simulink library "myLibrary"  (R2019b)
settings: Solver=VariableStepAuto  StartTime=0.0  StopTime=10.0  RelTol=1e-3
undefined symbols (not defined in the file or in its folder): batt_delay, Calculation, cap_1ph, cap_3ph, Complex, Current, Dynamic, EV, ev_charger, EV_ID, ev_num, gcbh, Iabc, Load, max_charge_1ph, max_charge_3ph, max_disch_1ph, max_disch_3ph, MV_LV_transf, myLibrary, phase, Phase, Phasor, rated_1ph, rated_3ph, Single, SoC_init, SPDL, sps_rtmsupport, Tr_capacity, Tstep, Vabc, Vnom, yes
libraries: powerlib x163, $bdroot x13, spsVIMeasurementModel x3, simulink x2, powerlib_meascontrol x1
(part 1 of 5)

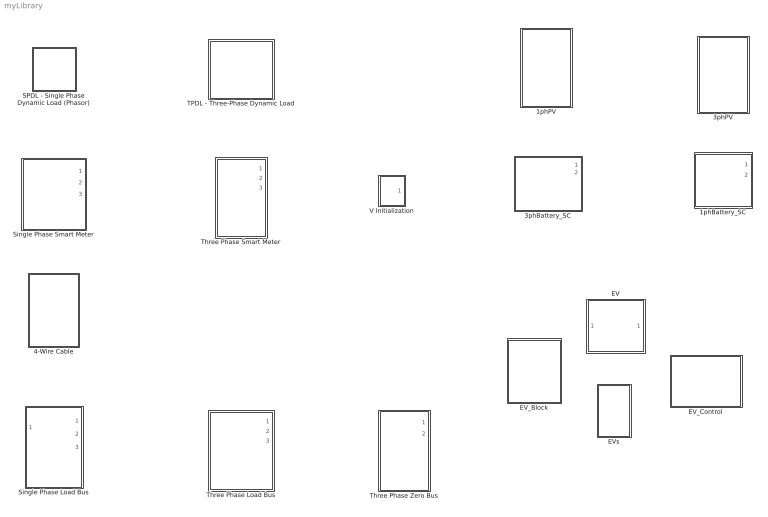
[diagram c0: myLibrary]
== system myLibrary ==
  1phBattery_SC : Subsystem  mask{Ecap=cap_1ph, Sn=rated_1ph, SoC=SoC_init, Pch_max=max_charge_1ph, Pdisc_max=max_disch_1ph, ch_delay=batt_delay, Phase=phase}
      mask prompts: Ecap "Capacity [kWh]"; Sn "Rated power [kVA]"; SoC "Initial SoC [%]"; Pch_max "Max charging rate [kW]"; Pdisc_max "Max discharge rate [kW]"; ch_delay "Charging delay [give integer multiple of time step]"; Phase "Connected Phase [1,2,3]"
      mask help: A 3phase battery system operating at 'self-consumption' mode
  1phPV : Subsystem  mask{Load_Profile=0, Phase=0, Capacity=0}
      mask prompts: Load_Profile "PV Profile"; Phase "Phase (A=1, B=2, C=3)"; Capacity "Capacity [kWp]"
  3phBattery_SC : Subsystem  mask{Ecap=cap_3ph, Sn=rated_3ph, SoC=SoC_init, Pch_max=max_charge_3ph, Pdisc_max=max_disch_3ph, ch_delay=batt_delay}
      mask prompts: Ecap "Capacity [kWh]"; Sn "Rated power [kVA]"; SoC "Initial SoC [%]"; Pch_max "Max charging rate [kW]"; Pdisc_max "Max discharge rate [kW]"; ch_delay "Charging delay [give integer multiple of time step]"
      mask help: A 3phase battery system operating at 'self-consumption' mode
  3phPV : Subsystem  mask{Load_Profile=0, Capacity=0}
      mask prompts: Load_Profile "PV Profile"; Capacity "Capacity [kWp]"
  4-Wire Cable : Subsystem  AncestorBlock=myLibrary/Three Phase Smart Meter  mask{R=0, L=0, C=0, Length=0}
      mask prompts: Length "Length (km)"
  EV : Subsystem  AncestorBlock=myLibrarya/EV  mask{Phase=1, EV_id=EV_ID}
      mask prompts: Phase "Connected Phase [1,2,3]"; EV_id "EV ID"
      mask help: Single Phase EV
  EV_Block : Subsystem  AncestorBlock=myLibrary/EV_Block  InitFcn=|
      | EV_num=20
      | Phase=[5,5,10];
      | ID_first_EV=1;
  EV_Control : Subsystem  AncestorBlock=myLibrary/EV_Control  InitFcn=ev_control_init
  EVs : Subsystem  mask{EV_ID=18, Phase=1}
      mask prompts: EV_ID "EV ID"
      mask init:
      | data_EV=sprintf('EV_num_%d',EV_ID);
      | set_param([gcb '/EVinfo'],'GotoTag',data_EV);
      | 
      | data_EV=sprintf('EV_cont_%d',EV_ID);
      | set_param([gcb '/EVcont'],'GotoTag',data_EV);
  SPDL - Single Phase Dynamic Load (Phasor) : Subsystem  mask(Single-Phase Dynamic Load){Load_Profile=0, Phase=0}
      mask prompts: Phase "Phase [A=1, B=2, C=3]"
      mask help: Single Phase Dynamic Load. The Load Profile is given by an external file.
  Single Phase Load Bus : Subsystem
  Single Phase Smart Meter : Subsystem
  TPDL - Three-Phase Dynamic Load : Subsystem  mask{Load_Profile=0}
  Three Phase Load Bus : Subsystem
  Three Phase Smart Meter : Subsystem
  Three Phase Zero Bus : Subsystem
  V Initialization : Subsystem

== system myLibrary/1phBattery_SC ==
  Constant7 : Constant  Value=0
  Pbatt_SoC : Subsystem
  SPDL2 : Subsystem  mask(Single-Phase Dynamic Load){Phase=Phase}
      mask prompts: Phase "Phase [A=1, B=2, C=3]"
      mask help: Single Phase Dynamic Load. The Load Profile is given by an external file.
  Single Phase Smart Meter : Subsystem
  P : PMIOPort  Tag=PMCPort  Side=Left
  N : PMIOPort  Tag=PMCPort  Port=2  Side=Left
  p : PMIOPort  Port=3  Side=Right
  n : PMIOPort  Port=4  Side=Right
  Pbatt : Outport
  SoC : Outport  Port=2
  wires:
  Constant7/1 -> [Q]
  [Q] -> SPDL2/2(Q)
  [P] -> SPDL2/1(P)
  Single Phase Smart Meter/1(Pout) -> [Pnet]
  [Pnet] -> Pbatt_SoC/1(Pn)
  Pbatt_SoC/1(SoC) -> SoC/1
  Pbatt_SoC/2(Pbatt) -> [P], Pbatt/1
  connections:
  p/RConn1 -- Single Phase Smart Meter/RConn1
  n/RConn1 -- Single Phase Smart Meter/RConn2
  P/RConn1 -- SPDL2/LConn1 -- Single Phase Smart Meter/LConn1
  N/RConn1 -- Single Phase Smart Meter/LConn2 -- SPDL2/LConn2

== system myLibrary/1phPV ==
  1Ph PV : $bdroot/3phPV/1Ph PV  Load_Profile=Load_Profile  Phase=Phase  Capacity=Capacity
  Voltage Measurement1 : powerlib/Measurements/Voltage Measurement  PhasorSimulation=off  OutputType=Complex  PSBequivalent=0
  Phase : PMIOPort  Tag=PMCPort  Side=Left
  N : PMIOPort  Tag=PMCPort  Port=2  Side=Left
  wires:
  Voltage Measurement1/1 -> 1Ph PV/1
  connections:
  Phase/RConn1 -- Voltage Measurement1/LConn1 -- 1Ph PV/LConn1
  N/RConn1 -- Voltage Measurement1/LConn2 -- 1Ph PV/LConn2

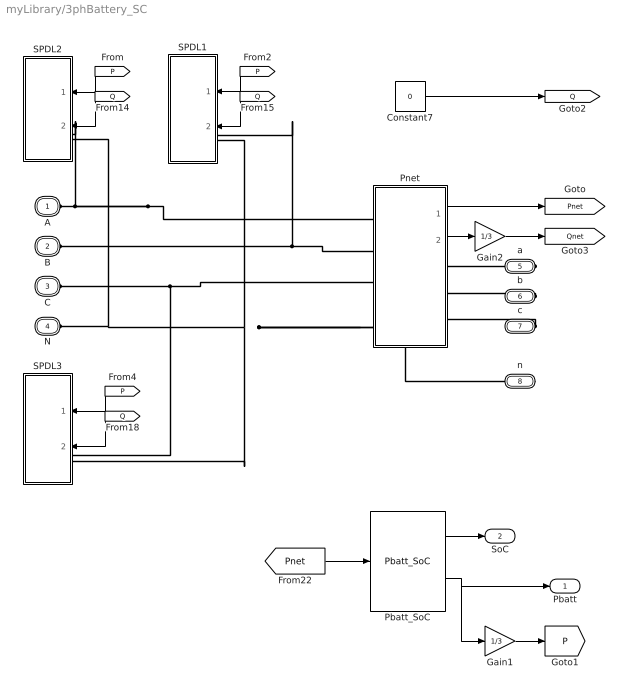
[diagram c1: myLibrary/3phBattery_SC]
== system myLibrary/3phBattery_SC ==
  Constant7 : Constant  Value=0
  Gain1 : Gain  Gain=1/3
  Gain2 : Gain  Gain=1/3
  Pbatt_SoC : $bdroot/1phBattery_SC/Pbatt_SoC  SystemSampleTime=-1  Latency=0  AutoFrameSizeCalculation=off
  Pnet : Subsystem
  SPDL1 : Subsystem  mask(Single-Phase Dynamic Load){Phase=2}
      mask prompts: Phase "Phase [A=1, B=2, C=3]"
      mask help: Single Phase Dynamic Load. The Load Profile is given by an external file.
  SPDL2 : Subsystem  mask(Single-Phase Dynamic Load){Phase=1}
      mask prompts: Phase "Phase [A=1, B=2, C=3]"
      mask help: Single Phase Dynamic Load. The Load Profile is given by an external file.
  SPDL3 : Subsystem  mask(Single-Phase Dynamic Load){Phase=3}
      mask prompts: Phase "Phase [A=1, B=2, C=3]"
      mask help: Single Phase Dynamic Load. The Load Profile is given by an external file.
  A : PMIOPort  Tag=PMCPort  Side=Left
  B : PMIOPort  Tag=PMCPort  Port=2  Side=Left
  C : PMIOPort  Tag=PMCPort  Port=3  Side=Left
  N : PMIOPort  Tag=PMCPort  Port=4  Side=Left
  a : PMIOPort  Port=5  Side=Right
  b : PMIOPort  Port=6  Side=Right
  c : PMIOPort  Port=7  Side=Right
  n : PMIOPort  Port=8  Side=Right
  Pbatt : Outport
  SoC : Outport  Port=2
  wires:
  [P] -> SPDL3/1(P)
  [Q] -> SPDL3/2(Q)
  [Q] -> SPDL2/2(Q)
  Gain2/1 -> [Qnet]
  [P] -> SPDL2/1(P)
  Pnet/1(Pnet) -> [Pnet]
  Constant7/1 -> [Q]
  [Pnet] -> Pbatt_SoC/1
  Gain1/1 -> [P]
  Pbatt_SoC/1 -> SoC/1
  Pbatt_SoC/2 -> Pbatt/1, Gain1/1
  [P] -> SPDL1/1(P)
  [Q] -> SPDL1/2(Q)
  Pnet/2(Qnet) -> Gain2/1
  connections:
  c/RConn1 -- Pnet/RConn3
  b/RConn1 -- Pnet/RConn2
  Pnet/RConn1 -- a/RConn1
  N/RConn1 -- SPDL2/LConn2 -- Pnet/LConn4 -- n/RConn1 -- SPDL3/LConn2 -- SPDL1/LConn2
  B/RConn1 -- SPDL1/LConn1 -- Pnet/LConn2
  C/RConn1 -- Pnet/LConn3 -- SPDL3/LConn1
  A/RConn1 -- SPDL2/LConn1 -- Pnet/LConn1

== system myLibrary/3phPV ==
  1Ph PV : Subsystem  mask{Load_Profile=Load_Profile, Phase=1, Capacity=Capacity/3}
      mask prompts: Load_Profile "PV Profile"; Capacity "Capacity [kWp]"
  1Ph PV1 : $bdroot/3phPV/1Ph PV  Load_Profile=Load_Profile  Phase=2  Capacity=Capacity/3
  1Ph PV2 : $bdroot/3phPV/1Ph PV  Load_Profile=Load_Profile  Phase=3  Capacity=Capacity/3
  Ground2 : powerlib/Elements/Ground  LConnTagsString=a
  Voltage Measurement : powerlib/Measurements/Voltage Measurement  PhasorSimulation=off  OutputType=Complex  PSBequivalent=0
  Voltage Measurement1 : powerlib/Measurements/Voltage Measurement  PhasorSimulation=off  OutputType=Complex  PSBequivalent=0
  Voltage Measurement2 : powerlib/Measurements/Voltage Measurement  PhasorSimulation=off  OutputType=Complex  PSBequivalent=0
  A : PMIOPort  Tag=PMCPort  Side=Left
  B : PMIOPort  Tag=PMCPort  Port=2  Side=Left
  C : PMIOPort  Tag=PMCPort  Port=3  Side=Left
  N : PMIOPort  Tag=PMCPort  Port=4  Side=Left
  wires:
  Voltage Measurement2/1 -> 1Ph PV/1(Vp)
  Voltage Measurement/1 -> 1Ph PV1/1
  Voltage Measurement1/1 -> 1Ph PV2/1
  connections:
  1Ph PV1/LConn2 -- 1Ph PV/LConn2 -- 1Ph PV2/LConn2 -- N/RConn1
  Voltage Measurement1/LConn1 -- 1Ph PV2/LConn1 -- C/RConn1
  Voltage Measurement/LConn1 -- 1Ph PV1/LConn1 -- B/RConn1
  Voltage Measurement2/LConn1 -- 1Ph PV/LConn1 -- A/RConn1
  Ground2/LConn1 -- Voltage Measurement1/LConn2 -- Voltage Measurement/LConn2 -- Voltage Measurement2/LConn2

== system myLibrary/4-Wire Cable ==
  Cag : powerlib/Elements/Series RLC Branch  LConnTagsString=__new0  RConnTagsString=__new0  BranchType=C  Resistance=1  Inductance=1e-3  SetiL0=off  InitialCurrent=0  Capacitance=C(1,1)*Length/2  Setx0=off  InitialVoltage=0  Measurements=None
  Cag1 : powerlib/Elements/Series RLC Branch  LConnTagsString=__new0  RConnTagsString=__new0  BranchType=C  Resistance=1  Inductance=1e-3  SetiL0=off  InitialCurrent=0  Capacitance=C(1,1)*Length/2  Setx0=off  InitialVoltage=0  Measurements=None
  Cbg : powerlib/Elements/Series RLC Branch  LConnTagsString=__new0  RConnTagsString=__new0  BranchType=C  Resistance=1  Inductance=1e-3  SetiL0=off  InitialCurrent=0  Capacitance=C(1,1)*Length/2  Setx0=off  InitialVoltage=0  Measurements=None
  Cbg1 : powerlib/Elements/Series RLC Branch  LConnTagsString=__new0  RConnTagsString=__new0  BranchType=C  Resistance=1  Inductance=1e-3  SetiL0=off  InitialCurrent=0  Capacitance=C(1,1)*Length/2  Setx0=off  InitialVoltage=0  Measurements=None
  Ccg : powerlib/Elements/Series RLC Branch  LConnTagsString=__new0  RConnTagsString=__new0  BranchType=C  Resistance=1  Inductance=1e-3  SetiL0=off  InitialCurrent=0  Capacitance=C(1,1)*Length/2  Setx0=off  InitialVoltage=0  Measurements=None
  Ccg1 : powerlib/Elements/Series RLC Branch  LConnTagsString=__new0  RConnTagsString=__new0  BranchType=C  Resistance=1  Inductance=1e-3  SetiL0=off  InitialCurrent=0  Capacitance=C(1,1)*Length/2  Setx0=off  InitialVoltage=0  Measurements=None
  Cng : powerlib/Elements/Series RLC Branch  LConnTagsString=__new0  RConnTagsString=__new0  BranchType=C  Resistance=1  Inductance=1e-3  SetiL0=off  InitialCurrent=0  Capacitance=C(2,1)*Length/2  Setx0=off  InitialVoltage=0  Measurements=None
  Cng1 : powerlib/Elements/Series RLC Branch  LConnTagsString=__new0  RConnTagsString=__new0  BranchType=C  Resistance=1  Inductance=1e-3  SetiL0=off  InitialCurrent=0  Capacitance=C(2,1)*Length/2  Setx0=off  InitialVoltage=0  Measurements=None
  Ground1 : powerlib/Elements/Ground  LConnTagsString=a
  Ground2 : powerlib/Elements/Ground  LConnTagsString=a
  Mutual Inductance : powerlib/Elements/Mutual Inductance  LConnTagsString=a|b|c|L4  RConnTagsString=A|B|C|R4  TypeOfMutual=Generalized mutual inductance  NumberOfWindings=4  SelfImpedance1=[1.1 1.1e-03]  SelfImpedance2=[ 1.1 1.1e-03]  ThreeWindings=on  SelfImpedance3=[ 1.1 1.1e-03]  MutualImpedance=[1.0 1.0e-03]  InductanceMatrix=L*Length  ResistanceMatrix=R*Length  Measurements=None
  A : PMIOPort  Side=Left
  B : PMIOPort  Port=2  Side=Left
  C : PMIOPort  Port=3  Side=Left
  N : PMIOPort  Port=4  Side=Left
  a : PMIOPort  Port=5  Side=Right
  b : PMIOPort  Port=6  Side=Right
  c : PMIOPort  Port=7  Side=Right
  n : PMIOPort  Port=8  Side=Right
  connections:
  A/RConn1 -- Mutual Inductance/LConn1 -- Cag/LConn1
  Mutual Inductance/RConn1 -- Cag1/LConn1 -- a/RConn1
  B/RConn1 -- Cbg/LConn1 -- Mutual Inductance/LConn2
  Mutual Inductance/RConn2 -- Cbg1/LConn1 -- b/RConn1
  C/RConn1 -- Ccg/LConn1 -- Mutual Inductance/LConn3
  c/RConn1 -- Ccg1/LConn1 -- Mutual Inductance/RConn3
  N/RConn1 -- Cng/LConn1 -- Mutual Inductance/LConn4
  n/RConn1 -- Cng1/LConn1 -- Mutual Inductance/RConn4
  Cag/RConn1 -- Ground2/LConn1 -- Cng/RConn1 -- Ccg/RConn1 -- Cbg/RConn1
  Cag1/RConn1 -- Ground1/LConn1 -- Cng1/RConn1 -- Ccg1/RConn1 -- Cbg1/RConn1

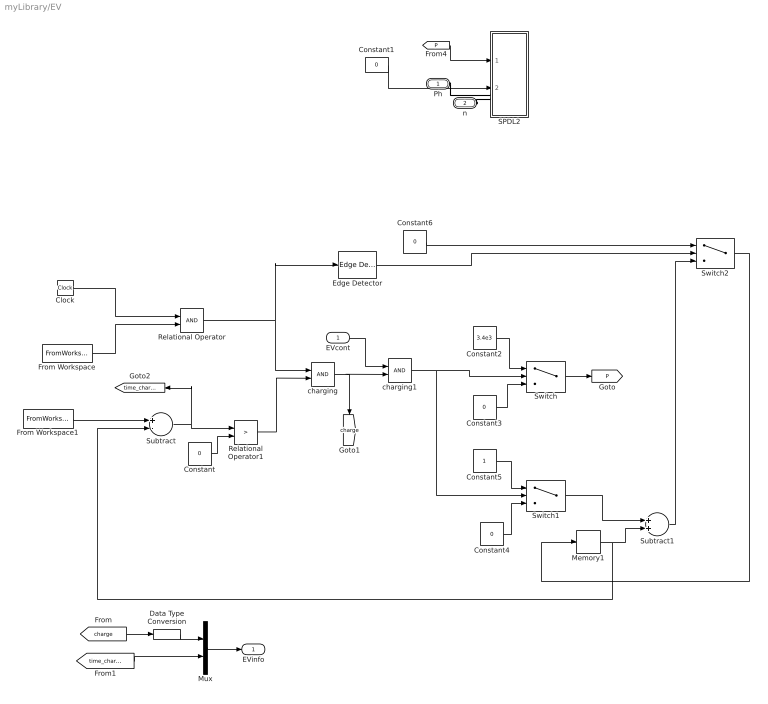
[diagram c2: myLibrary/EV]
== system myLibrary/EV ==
  EVcont : Inport
  Clock : Clock
  Constant{,1,3..4,6} (5 alike) : Constant  Value=0
  Constant2 : Constant  Value=3.4e3
  Constant5 : Constant
  Data Type Conversion : DataTypeConversion  OutDataTypeStr=double
  Edge Detector : powerlib_meascontrol/Logic/Edge Detector  model=Falling  ic=0  Ts=0
  From Workspace : FromWorkspace  VariableName=ch_t(EV_id)  Interpolate=off  OutputAfterFinalValue=Holding final value
  From Workspace1 : FromWorkspace  VariableName=needed_time_ch(EV_id)  Interpolate=off  OutputAfterFinalValue=Holding final value
  Memory1 : Memory
  Mux : Mux  Inputs=2
  Relational Operator : RelationalOperator  OutDataTypeStr=boolean  RndMeth=Simplest
  Relational Operator1 : RelationalOperator  Operator=>  OutDataTypeStr=boolean  RndMeth=Simplest
  SPDL2 : Subsystem  AncestorBlock=myLibrary/SPDL - Single Phase Dynamic Load (Phasor)  mask(Single-Phase Dynamic Load){Phase=Phase}
      mask prompts: Phase "Phase [A=1, B=2, C=3]"
      mask help: Single Phase Dynamic Load. The Load Profile is given by an external file.
  Subtract : Sum  Inputs=+-
  Subtract1 : Sum
  Switch : Switch  Criteria=u2 > Threshold
  Switch1 : Switch  Criteria=u2 > Threshold
  Switch2 : Switch  Criteria=u2 > Threshold
  charging : Logic  AllPortsSameDT=off  OutDataTypeStr=boolean
  charging1 : Logic  AllPortsSameDT=off  OutDataTypeStr=boolean
  Ph : PMIOPort  Side=Left
  n : PMIOPort  Port=2  Side=Left
  EVinfo : Outport
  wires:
  Data Type Conversion/1 -> Mux/1
  EVcont/1 -> charging1/1
  charging1/1 -> Switch/2, Switch1/2
  Mux/1 -> EVinfo/1
  [time_charge] -> Mux/2
  [charge] -> Data Type Conversion/1
  Switch2/1 -> Memory1/1
  Subtract1/1 -> Switch2/3
  Constant6/1 -> Switch2/1
  Edge Detector/1 -> Switch2/2
  Memory1/1 -> Subtract1/2, Subtract/2
  Switch1/1 -> Subtract1/1
  Constant5/1 -> Switch1/1
  Constant4/1 -> Switch1/3
  Switch/1 -> [P]
  Constant1/1 -> SPDL2/2(Q)
  [P] -> SPDL2/1(P)
  Constant3/1 -> Switch/3
  Constant2/1 -> Switch/1
  charging/1 -> [charge], charging1/2
  Relational Operator1/1 -> charging/2
  Relational Operator/1 -> charging/1, Edge Detector/1
  From Workspace1/1 -> Subtract/1
  Constant/1 -> Relational Operator1/2
  Subtract/1 -> Relational Operator1/1, [time_charge]
  From Workspace/1 -> Relational Operator/2
  Clock/1 -> Relational Operator/1
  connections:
  n/RConn1 -- SPDL2/LConn2
  Ph/RConn1 -- SPDL2/LConn1

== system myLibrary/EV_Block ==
  Block_EVs : Subsystem  InitFcn=ev_block_init
  A : PMIOPort  Tag=PMCPort  Side=Left
  B : PMIOPort  Tag=PMCPort  Port=2  Side=Left
  C : PMIOPort  Tag=PMCPort  Port=3  Side=Left
  N : PMIOPort  Tag=PMCPort  Port=4  Side=Left
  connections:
  A/RConn1 -- Block_EVs/LConn1
  B/RConn1 -- Block_EVs/LConn2
  C/RConn1 -- Block_EVs/LConn3
  N/RConn1 -- Block_EVs/LConn4

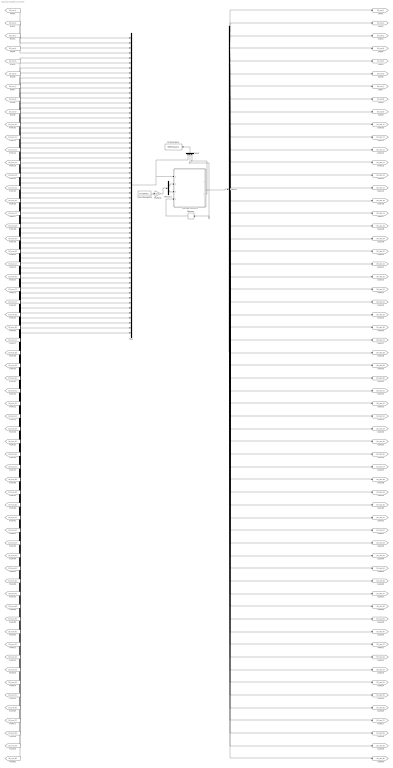
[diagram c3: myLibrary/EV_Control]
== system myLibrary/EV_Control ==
  Demux : Demux  Outputs=ev_num
  Demux1 : Demux  Outputs=2
  From Workspace : FromWorkspace  VariableName=Total_S  SampleTime=0  Interpolate=off  OutputAfterFinalValue=Holding final value
  MATLAB Function : MATLAB Function  TreatAsAtomicUnit=on
  Memory : Memory
  Multiply : Gain  Gain=1/1e3
  Mux : Mux  Inputs=ev_num
  Mux2 : Mux  Inputs=3
  To Workspace : ToWorkspace  VariableName=EVsignals  SaveFormat=Structure With Time  SampleTime=-1
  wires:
  From Workspace/1 -> Multiply/1
  Mux/1 -> MATLAB Function/1(EVsignals), Mux2/1
  MATLAB Function/1(EV_cont_signals) -> Memory/1, Demux/1, Mux2/2
  MATLAB Function/2(k) -> Mux2/3
  Mux2/1 -> To Workspace/1
  Memory/1 -> MATLAB Function/4(were_charging)
  Multiply/1 -> Demux1/1
  Demux1/1 -> MATLAB Function/2(P)
  Demux1/2 -> MATLAB Function/3(Q)
  [EV_num_1] -> Mux/1
  Demux/1 -> [EV_cont_1]
  [EV_num_2] -> Mux/2
  Demux/2 -> [EV_cont_2]
  [EV_num_3] -> Mux/3
  Demux/3 -> [EV_cont_3]
  [EV_num_4] -> Mux/4
  Demux/4 -> [EV_cont_4]
  [EV_num_5] -> Mux/5
  Demux/5 -> [EV_cont_5]
  [EV_num_6] -> Mux/6
  Demux/6 -> [EV_cont_6]
  [EV_num_7] -> Mux/7
  Demux/7 -> [EV_cont_7]
  [EV_num_8] -> Mux/8
  Demux/8 -> [EV_cont_8]
  [EV_num_9] -> Mux/9
  Demux/9 -> [EV_cont_9]
  [EV_num_10] -> Mux/10
  Demux/10 -> [EV_cont_10]
  [EV_num_11] -> Mux/11
  Demux/11 -> [EV_cont_11]
  [EV_num_12] -> Mux/12
  Demux/12 -> [EV_cont_12]
  [EV_num_13] -> Mux/13
  Demux/13 -> [EV_cont_13]
  [EV_num_14] -> Mux/14
  Demux/14 -> [EV_cont_14]
  [EV_num_15] -> Mux/15
  Demux/15 -> [EV_cont_15]
  [EV_num_16] -> Mux/16
  Demux/16 -> [EV_cont_16]
  [EV_num_17] -> Mux/17
  Demux/17 -> [EV_cont_17]
  [EV_num_18] -> Mux/18
  Demux/18 -> [EV_cont_18]
  [EV_num_19] -> Mux/19
  Demux/19 -> [EV_cont_19]
  [EV_num_20] -> Mux/20
  Demux/20 -> [EV_cont_20]
  [EV_num_21] -> Mux/21
  Demux/21 -> [EV_cont_21]
  [EV_num_22] -> Mux/22
  Demux/22 -> [EV_cont_22]
  [EV_num_23] -> Mux/23
  Demux/23 -> [EV_cont_23]
  [EV_num_24] -> Mux/24
  Demux/24 -> [EV_cont_24]
  [EV_num_25] -> Mux/25
  Demux/25 -> [EV_cont_25]
  [EV_num_26] -> Mux/26
  Demux/26 -> [EV_cont_26]
  [EV_num_27] -> Mux/27
  Demux/27 -> [EV_cont_27]
  [EV_num_28] -> Mux/28
  Demux/28 -> [EV_cont_28]
  [EV_num_29] -> Mux/29
  Demux/29 -> [EV_cont_29]
  [EV_num_30] -> Mux/30
  Demux/30 -> [EV_cont_30]
  [EV_num_31] -> Mux/31
  Demux/31 -> [EV_cont_31]
  [EV_num_32] -> Mux/32
  Demux/32 -> [EV_cont_32]
  [EV_num_33] -> Mux/33
  Demux/33 -> [EV_cont_33]
  [EV_num_34] -> Mux/34
  Demux/34 -> [EV_cont_34]
  [EV_num_35] -> Mux/35
  Demux/35 -> [EV_cont_35]
  [EV_num_36] -> Mux/36
  Demux/36 -> [EV_cont_36]
  [EV_num_37] -> Mux/37
  Demux/37 -> [EV_cont_37]
  [EV_num_38] -> Mux/38
  Demux/38 -> [EV_cont_38]
  [EV_num_39] -> Mux/39
  Demux/39 -> [EV_cont_39]
  [EV_num_40] -> Mux/40
  Demux/40 -> [EV_cont_40]
  [EV_num_41] -> Mux/41
  Demux/41 -> [EV_cont_41]
  [EV_num_42] -> Mux/42
  Demux/42 -> [EV_cont_42]
  [EV_num_43] -> Mux/43
  Demux/43 -> [EV_cont_43]
  [EV_num_44] -> Mux/44
  Demux/44 -> [EV_cont_44]
  [EV_num_45] -> Mux/45
  Demux/45 -> [EV_cont_45]
  [EV_num_46] -> Mux/46
  Demux/46 -> [EV_cont_46]
  [EV_num_47] -> Mux/47
  Demux/47 -> [EV_cont_47]
  [EV_num_48] -> Mux/48
  Demux/48 -> [EV_cont_48]
  [EV_num_49] -> Mux/49
  Demux/49 -> [EV_cont_49]
  [EV_num_50] -> Mux/50
  Demux/50 -> [EV_cont_50]
  [EV_num_51] -> Mux/51
  Demux/51 -> [EV_cont_51]
  [EV_num_52] -> Mux/52
  Demux/52 -> [EV_cont_52]
  [EV_num_53] -> Mux/53
  Demux/53 -> [EV_cont_53]
  [EV_num_54] -> Mux/54
  Demux/54 -> [EV_cont_54]
  [EV_num_55] -> Mux/55
  Demux/55 -> [EV_cont_55]
  [EV_num_56] -> Mux/56
  Demux/56 -> [EV_cont_56]
  [EV_num_57] -> Mux/57
  Demux/57 -> [EV_cont_57]
  [EV_num_58] -> Mux/58
  Demux/58 -> [EV_cont_58]
  [EV_num_59] -> Mux/59
  Demux/59 -> [EV_cont_59]
  [EV_num_60] -> Mux/60
  Demux/60 -> [EV_cont_60]

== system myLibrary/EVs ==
  EV2 : $bdroot/EV  Phase=Phase  EV_id=EV_ID
  Ph : PMIOPort  Side=Left
  n : PMIOPort  Port=2  Side=Left
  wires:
  [EV_cont_18] -> EV2/1
  EV2/1 -> [EV_num_18]
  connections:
  EV2/LConn1 -- Ph/RConn1
  EV2/LConn2 -- n/RConn1

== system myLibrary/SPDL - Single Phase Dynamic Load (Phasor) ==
  Breaker : powerlib/Elements/Breaker  InitialState=1  SwitchingTimes=0  External=off  BreakerResistance=0.01  SnubberResistance=1e3  SnubberCapacitance=inf  Measurements=None  MoreParameters=on  NoBreakLoop=off
  Controlled Current Source : powerlib/Electrical Sources/Controlled Current Source  Initialize=on  Source_Type=AC  Amplitude=0  Phase=0  Frequency=50  Measurements=None
  Current Calculation : Subsystem
  Gain : Gain  Gain=sqrt(2)
  Snubber4 : powerlib/Elements/Series RLC Branch  LConnTagsString=__new0  RConnTagsString=__new0  BranchType=R  Resistance=1e6  Inductance=1e-3  SetiL0=off  InitialCurrent=0  Capacitance=1e-6  Setx0=off  InitialVoltage=0  Measurements=None
  Step : Step  Time=0.001  Before=-1  SampleTime=0
  Switch : Switch  Criteria=u2 > Threshold
  V Initialization : $bdroot/V Initialization  SystemSampleTime=-1  Latency=0  AutoFrameSizeCalculation=off
  Voltage Measurement : powerlib/Measurements/Voltage Measurement  PhasorSimulation=off  OutputType=Complex  PSBequivalent=0
  Phase : PMIOPort  Side=Left
  Neutral : PMIOPort  Port=2  Side=Left
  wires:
  Voltage Measurement/1 -> [Vm_c]
  Switch/1 -> Current Calculation/1(Vp)
  Current Calculation/1(Isignal) -> [Icontrol]
  [Icontrol] -> Controlled Current Source/1
  [Vm_c] -> Switch/1
  V Initialization/1 -> Gain/1
  Step/1 -> Switch/2
  Gain/1 -> Switch/3
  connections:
  Voltage Measurement/LConn2 -- Snubber4/RConn1 -- Controlled Current Source/RConn1 -- Neutral/RConn1
  Controlled Current Source/LConn1 -- Breaker/RConn1 -- Voltage Measurement/LConn1 -- Phase/RConn1
  Snubber4/LConn1 -- Breaker/LConn1

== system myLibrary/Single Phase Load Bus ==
  Ph : Inport
  Complex to Magnitude-Angle : ComplexToMagnitudeAngle
  Complex to Magnitude-Angle1 : ComplexToMagnitudeAngle
  Mux3 : Mux  Inputs=2
  Mux4 : Mux  Inputs=2
  Rad->Deg. : Gain  Gain=1/sqrt(2)
  Rad->Deg.1 : Gain  Gain=1/sqrt(2)
  Rad->Deg.2 : Gain  Gain=180/pi
  Rad->Deg.3 : Gain  Gain=180/pi
  Single Phase Smart Meter : $bdroot/Single Phase Smart Meter  SystemSampleTime=-1  Latency=0  AutoFrameSizeCalculation=off
  Subsystem : Subsystem
  Phase : PMIOPort  Tag=PMCPort  Side=Left
  N : PMIOPort  Tag=PMCPort  Port=2  Side=Left
  phase : PMIOPort  Tag=PMCPort  Port=3  Side=Right
  n : PMIOPort  Tag=PMCPort  Port=4  Side=Right
  Vnode : Outport  VectorParamsAs1DForOutWhenUnconnected=off
  Inode : Outport  Port=2  VectorParamsAs1DForOutWhenUnconnected=off
  Lmeas : Outport  Port=3  VectorParamsAs1DForOutWhenUnconnected=off
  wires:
  Single Phase Smart Meter/1 -> Subsystem/1(Vpn)
  Complex to Magnitude-Angle/1 -> Rad->Deg./1
  Rad->Deg.2/1 -> Mux4/2
  Rad->Deg.3/1 -> Mux3/2
  Rad->Deg.1/1 -> Mux3/1
  Complex to Magnitude-Angle1/1 -> Rad->Deg.1/1
  Rad->Deg./1 -> Mux4/1
  Mux4/1 -> Vnode/1
  Subsystem/2("I_pn ") -> Complex to Magnitude-Angle1/1
  Complex to Magnitude-Angle1/2 -> Rad->Deg.3/1
  Complex to Magnitude-Angle/2 -> Rad->Deg.2/1
  Mux3/1 -> Inode/1
  Subsystem/1(V_pn) -> Complex to Magnitude-Angle/1
  Single Phase Smart Meter/2 -> Subsystem/2(Ipn)
  Single Phase Smart Meter/3 -> Lmeas/1
  Ph/1 -> Subsystem/3(Ph)
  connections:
  Phase/RConn1 -- Single Phase Smart Meter/LConn1
  N/RConn1 -- Single Phase Smart Meter/LConn2
  phase/RConn1 -- Single Phase Smart Meter/RConn1
  Single Phase Smart Meter/RConn2 -- n/RConn1

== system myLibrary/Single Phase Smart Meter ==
  Meas : Subsystem
  Phase-Ground Measurements : Subsystem
  Phase-Neutral Measurements : Subsystem
  Phase : PMIOPort  Side=Left
  Neutral : PMIOPort  Port=2  Side=Left
  phase : PMIOPort  Port=3  Side=Right
  neutral : PMIOPort  Port=4  Side=Right
  Vp_Vn : Outport  VectorParamsAs1DForOutWhenUnconnected=off
  Ip_In : Outport  Port=2  VectorParamsAs1DForOutWhenUnconnected=off
  Measurements : Outport  Port=3  VectorParamsAs1DForOutWhenUnconnected=off
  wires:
  Phase-Ground Measurements/2(Ip_In) -> Ip_In/1, Meas/2(Ipn)
  Meas/1(Measurements) -> Measurements/1
  Phase-Ground Measurements/1(Vp_Vn) -> Vp_Vn/1
  Phase-Neutral Measurements/1(Vpn) -> Meas/1(Vpn)
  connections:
  Phase-Ground Measurements/LConn1 -- Phase-Neutral Measurements/LConn1 -- Phase/RConn1
  Neutral/RConn1 -- Phase-Neutral Measurements/LConn2 -- Phase-Ground Measurements/LConn2
  phase/RConn1 -- Phase-Ground Measurements/RConn1
  neutral/RConn1 -- Phase-Ground Measurements/RConn2

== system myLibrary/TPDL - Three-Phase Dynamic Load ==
  SPDL - Single Phase Dynamic Load (Phasor) : Subsystem  mask(Single-Phase Dynamic Load){Load_Profile=Load_Profile, Phase=1}
      mask prompts: Phase "Phase [A=1, B=2, C=3]"
      mask help: Single Phase Dynamic Load. The Load Profile is given by an external file.
  SPDL - Single Phase Dynamic Load (Phasor)1 : Subsystem  mask(Single-Phase Dynamic Load){Load_Profile=Load_Profile, Phase=2}
      mask prompts: Phase "Phase [A=1, B=2, C=3]"
      mask help: Single Phase Dynamic Load. The Load Profile is given by an external file.
  SPDL - Single Phase Dynamic Load (Phasor)2 : Subsystem  mask(Single-Phase Dynamic Load){Load_Profile=Load_Profile, Phase=3}
      mask prompts: Phase "Phase [A=1, B=2, C=3]"
      mask help: Single Phase Dynamic Load. The Load Profile is given by an external file.
  A : PMIOPort  Side=Left
  B : PMIOPort  Port=2  Side=Left
  C : PMIOPort  Port=3  Side=Left
  N : PMIOPort  Port=4  Side=Left
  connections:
  A/RConn1 -- SPDL - Single Phase Dynamic Load (Phasor)/LConn1
  B/RConn1 -- SPDL - Single Phase Dynamic Load (Phasor)1/LConn1
  C/RConn1 -- SPDL - Single Phase Dynamic Load (Phasor)2/LConn1
  N/RConn1 -- SPDL - Single Phase Dynamic Load (Phasor)/LConn2 -- SPDL - Single Phase Dynamic Load (Phasor)1/LConn2 -- SPDL - Single Phase Dynamic Load (Phasor)2/LConn2

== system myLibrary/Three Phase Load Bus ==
  Complex to Magnitude-Angle : ComplexToMagnitudeAngle
  Complex to Magnitude-Angle1 : ComplexToMagnitudeAngle
  Mux3 : Mux  Inputs=2
  Mux4 : Mux  Inputs=2
  Rad->Deg. : Gain  Gain=1/sqrt(2)
  Rad->Deg.1 : Gain  Gain=1/sqrt(2)
  Rad->Deg.2 : Gain  Gain=180/pi
  Rad->Deg.3 : Gain  Gain=180/pi
  Three Phase Smart Meter : $bdroot/Three Phase Smart Meter  SystemSampleTime=-1  Latency=0  AutoFrameSizeCalculation=off
  A : PMIOPort  Tag=PMCPort  Side=Left
  B : PMIOPort  Tag=PMCPort  Port=2  Side=Left
  C : PMIOPort  Tag=PMCPort  Port=3  Side=Left
  N : PMIOPort  Tag=PMCPort  Port=4  Side=Left
  a : PMIOPort  Tag=PMCPort  Port=5  Side=Right
  b : PMIOPort  Tag=PMCPort  Port=6  Side=Right
  c : PMIOPort  Tag=PMCPort  Port=7  Side=Right
  n : PMIOPort  Tag=PMCPort  Port=8  Side=Right
  Vnode : Outport  VectorParamsAs1DForOutWhenUnconnected=off
  Inode : Outport  Port=2  VectorParamsAs1DForOutWhenUnconnected=off
  Lmeas : Outport  Port=3  VectorParamsAs1DForOutWhenUnconnected=off
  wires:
  Three Phase Smart Meter/3 -> Lmeas/1
  Complex to Magnitude-Angle1/1 -> Rad->Deg.1/1
  Complex to Magnitude-Angle1/2 -> Rad->Deg.3/1
  Complex to Magnitude-Angle/2 -> Rad->Deg.2/1
  Mux3/1 -> Inode/1
  Rad->Deg./1 -> Mux4/1
  Mux4/1 -> Vnode/1
  Rad->Deg.3/1 -> Mux3/2
  Rad->Deg.1/1 -> Mux3/1
  Rad->Deg.2/1 -> Mux4/2
  Complex to Magnitude-Angle/1 -> Rad->Deg./1
  Three Phase Smart Meter/1 -> Complex to Magnitude-Angle/1
  Three Phase Smart Meter/2 -> Complex to Magnitude-Angle1/1
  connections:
  A/RConn1 -- Three Phase Smart Meter/LConn1
  B/RConn1 -- Three Phase Smart Meter/LConn2
  C/RConn1 -- Three Phase Smart Meter/LConn3
  N/RConn1 -- Three Phase Smart Meter/LConn4
  a/RConn1 -- Three Phase Smart Meter/RConn1
  Three Phase Smart Meter/RConn2 -- b/RConn1
  Three Phase Smart Meter/RConn3 -- c/RConn1
  Three Phase Smart Meter/RConn4 -- n/RConn1

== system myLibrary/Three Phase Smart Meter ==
  Current Measurement : powerlib/Measurements/Current Measurement  PhasorSimulation=off  OutputType=Complex  PSBequivalent=0
  Ground1 : powerlib/Elements/Ground  LConnTagsString=a
  Mux : Mux  Inputs=2
  Mux1 : Mux  Inputs=2
  Mux2 : Mux  Inputs=3
  Three Phase Smart Meter : Subsystem
  Three-Phase V-I Measurement : Subsystem  AncestorBlock=powerlib/Measurements/Three-Phase V-I Measurement  DialogController=POWERSYS.PowerSysDialog  LoadFcn=|  StartFcn=sps_rtmsupport('StartFcn',gcbh);  StopFcn=sps_rtmsupport('StopFcn',gcbh);  mask(Three-Phase VI Measurement){VoltageMeasurement=phase-to-ground, SetLabelV=off, LabelV=Vabc, Vpu=off, VpuLL=off, CurrentMeasurement=yes, SetLabelI=off, LabelI=Iabc, Ipu=off, Pbase=100e6, Vbase=500e3, OutputType=Complex, PhasorSimulation=off, PSBequivalent=0}
      | if ~strcmp(get_param(bdroot,'BlockDiagramType'),'library')
      |     set_param([gcb,'/Model'],'LinkStatus','restore');
      | end
      | sps_rtmsupport('LoadFcn',gcbh);
      mask prompts: VoltageMeasurement "Voltage measurement"; SetLabelV "Use a label"; LabelV "Signal label  (use a From block to collect this signal)"; Vpu "Voltages in pu,  based on peak value of nominal phase-to-ground voltage"; VpuLL "Voltages in pu,  based on peak value of nominal phase-to-phase  voltage"; CurrentMeasurement "Current measurement"; SetLabelI "Use a label"; LabelI "Signal label  (use a From block to collect this signal)"; Ipu "Currents in pu"; Pbase "Base power ( VA 3 phase)"; Vbase "Nominal voltage used for pu measurement (Vrms phase-phase) :"; OutputType "Output signals in:"; PhasorSimulation "Phasor simulation (internal use)"; PSBequivalent "Equivalent circuit (internal use)"
      mask help: Ideal three-phase voltage and current measurements. The block can output the voltages and currents in per unit values or in volts and amperes.
      mask init:
      | block = gcb;
      | Kv=1;
      | Ki=1;
      | [Kv,Ki] = powericon('ThreePhaseVIMeasurementParam',block,Vpu,VpuLL,Ipu,Vbase,Pbase,PhasorSimulation,OutputType);
      | powericon('ThreePhaseVIMeasurementCback',block);
      | power_initmask();
  Voltage Measurement{1..4} (4 alike) : powerlib/Measurements/Voltage Measurement  PhasorSimulation=off  OutputType=Complex  PSBequivalent=0
  A : PMIOPort  Side=Left
  B : PMIOPort  Port=2  Side=Left
  C : PMIOPort  Port=3  Side=Left
  N : PMIOPort  Port=4  Side=Left
  a : PMIOPort  Port=5  Side=Right
  b : PMIOPort  Port=6  Side=Right
  c : PMIOPort  Port=7  Side=Right
  n : PMIOPort  Port=8  Side=Right
  Vabcn : Outport  VectorParamsAs1DForOutWhenUnconnected=off
  Iabcn : Outport  Port=2  VectorParamsAs1DForOutWhenUnconnected=off
  Meas. : Outport  Port=3  VectorParamsAs1DForOutWhenUnconnected=off
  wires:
  Mux/1 -> Vabcn/1
  Voltage Measurement3/1 -> Mux/2
  Three-Phase V-I Measurement/2(Iabc) -> Three Phase Smart Meter/2(Iabc), Mux1/1
  Three-Phase V-I Measurement/1(Vabc) -> Mux/1
  Three Phase Smart Meter/1(Meas.) -> Meas./1
  Current Measurement/1 -> Mux1/2
  Mux1/1 -> Iabcn/1
  Voltage Measurement2/1 -> Mux2/2
  Voltage Measurement1/1 -> Mux2/1
  Voltage Measurement4/1 -> Mux2/3
  Mux2/1 -> Three Phase Smart Meter/1(Vabc)
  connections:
  N/RConn1 -- Voltage Measurement4/LConn2 -- Voltage Measurement2/LConn2 -- Voltage Measurement1/LConn2 -- Voltage Measurement3/LConn1 -- Current Measurement/LConn1
  C/RConn1 -- Voltage Measurement4/LConn1 -- Three-Phase V-I Measurement/LConn3
  A/RConn1 -- Voltage Measurement1/LConn1 -- Three-Phase V-I Measurement/LConn1
  B/RConn1 -- Voltage Measurement2/LConn1 -- Three-Phase V-I Measurement/LConn2
  Voltage Measurement3/LConn2 -- Ground1/LConn1
  c/RConn1 -- Three-Phase V-I Measurement/RConn3
  b/RConn1 -- Three-Phase V-I Measurement/RConn2
  a/RConn1 -- Three-Phase V-I Measurement/RConn1
  Current Measurement/RConn1 -- n/RConn1

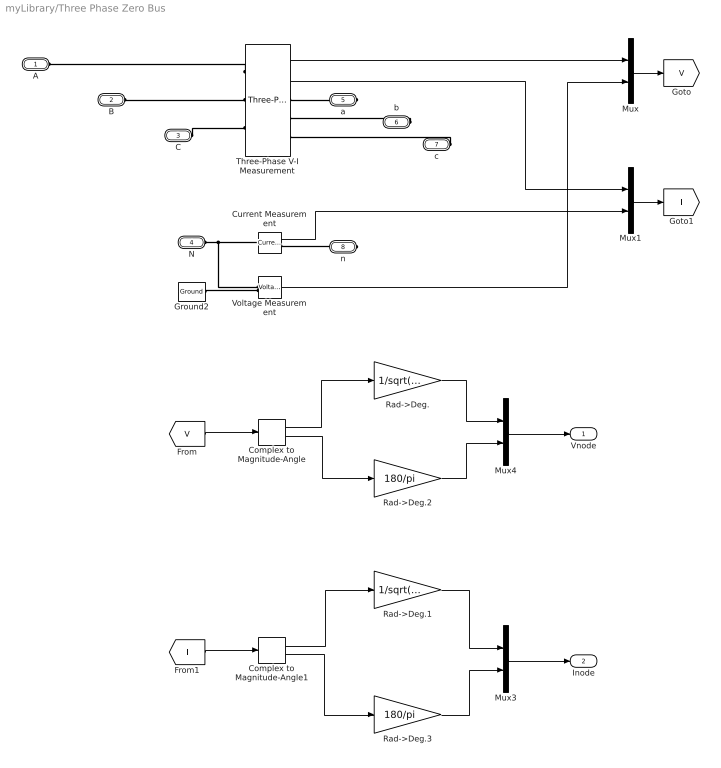
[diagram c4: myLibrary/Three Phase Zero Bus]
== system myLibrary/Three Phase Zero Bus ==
  Complex to Magnitude-Angle : ComplexToMagnitudeAngle
  Complex to Magnitude-Angle1 : ComplexToMagnitudeAngle
  Current Measurement : powerlib/Measurements/Current Measurement  PhasorSimulation=off  OutputType=Complex  PSBequivalent=0
  Ground2 : powerlib/Elements/Ground  LConnTagsString=a
  Mux{,1,3..4} (4 alike) : Mux  Inputs=2
  Rad->Deg. : Gain  Gain=1/sqrt(2)
  Rad->Deg.1 : Gain  Gain=1/sqrt(2)
  Rad->Deg.2 : Gain  Gain=180/pi
  Rad->Deg.3 : Gain  Gain=180/pi
  Three-Phase V-I Measurement : powerlib/Measurements/Three-Phase V-I Measurement  VoltageMeasurement=phase-to-ground  SetLabelV=off  LabelV=Vabc  Vpu=off  VpuLL=off  CurrentMeasurement=yes  SetLabelI=off  LabelI=Iabc  Ipu=off  Pbase=100e6  Vbase=500e3  OutputType=Complex  PhasorSimulation=off  PSBequivalent=0
  Voltage Measurement : powerlib/Measurements/Voltage Measurement  PhasorSimulation=off  OutputType=Complex  PSBequivalent=0
  A : PMIOPort  Side=Left
  B : PMIOPort  Port=2  Side=Left
  C : PMIOPort  Port=3  Side=Left
  N : PMIOPort  Port=4  Side=Left
  a : PMIOPort  Port=5  Side=Right
  b : PMIOPort  Port=6  Side=Right
  c : PMIOPort  Port=7  Side=Right
  n : PMIOPort  Port=8  Side=Right
  Vnode : Outport  VectorParamsAs1DForOutWhenUnconnected=off
  Inode : Outport  Port=2  VectorParamsAs1DForOutWhenUnconnected=off
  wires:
  Mux3/1 -> Inode/1
  Rad->Deg.1/1 -> Mux3/1
  Complex to Magnitude-Angle1/1 -> Rad->Deg.1/1
  Rad->Deg.3/1 -> Mux3/2
  Complex to Magnitude-Angle/2 -> Rad->Deg.2/1
  Rad->Deg./1 -> Mux4/1
  Complex to Magnitude-Angle/1 -> Rad->Deg./1
  Mux4/1 -> Vnode/1
  Rad->Deg.2/1 -> Mux4/2
  [V] -> Complex to Magnitude-Angle/1
  [I] -> Complex to Magnitude-Angle1/1
  Complex to Magnitude-Angle1/2 -> Rad->Deg.3/1
  Three-Phase V-I Measurement/1 -> Mux/1
  Voltage Measurement/1 -> Mux/2
  Mux/1 -> [V]
  Three-Phase V-I Measurement/2 -> Mux1/1
  Current Measurement/1 -> Mux1/2
  Mux1/1 -> [I]
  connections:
  Three-Phase V-I Measurement/LConn1 -- A/RConn1
  B/RConn1 -- Three-Phase V-I Measurement/LConn2
  C/RConn1 -- Three-Phase V-I Measurement/LConn3
  a/RConn1 -- Three-Phase V-I Measurement/RConn1
  b/RConn1 -- Three-Phase V-I Measurement/RConn2
  c/RConn1 -- Three-Phase V-I Measurement/RConn3
  N/RConn1 -- Current Measurement/LConn1 -- Voltage Measurement/LConn1
  n/RConn1 -- Current Measurement/RConn1
  Ground2/LConn1 -- Voltage Measurement/LConn2

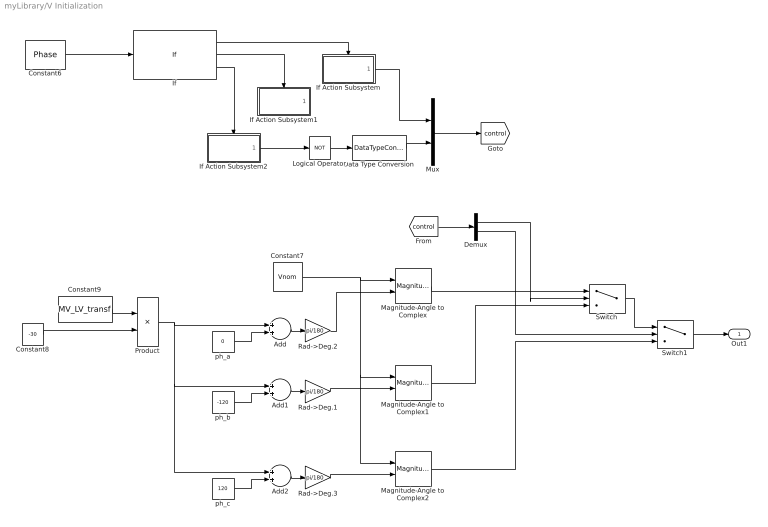
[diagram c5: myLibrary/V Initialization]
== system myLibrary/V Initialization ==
  Add : Sum
  Add1 : Sum
  Add2 : Sum
  Constant6 : Constant  Value=Phase
  Constant7 : Constant  Value=Vnom
  Constant8 : Constant  Value=-30
  Constant9 : Constant  Value=MV_LV_transf
  Data Type Conversion : DataTypeConversion  OutDataTypeStr=double
  Demux : Demux  Outputs=2
  If : If  IfExpression=u1 == 1  ElseIfExpressions=u1 == 2
  If Action Subsystem : Subsystem  TreatAsAtomicUnit=on
  If Action Subsystem1 : Subsystem  TreatAsAtomicUnit=on
  If Action Subsystem2 : Subsystem  TreatAsAtomicUnit=on
  Logical Operator : Logic  Operator=NOT  AllPortsSameDT=off  OutDataTypeStr=boolean
  Magnitude-Angle to Complex : MagnitudeAngleToComplex
  Magnitude-Angle to Complex1 : MagnitudeAngleToComplex
  Magnitude-Angle to Complex2 : MagnitudeAngleToComplex
  Mux : Mux  Inputs=2
  Product : Product
  Rad->Deg.1 : Gain  Gain=pi/180
  Rad->Deg.2 : Gain  Gain=pi/180
  Rad->Deg.3 : Gain  Gain=pi/180
  Switch : Switch  Criteria=u2 > Threshold
  Switch1 : Switch  Criteria=u2 > Threshold
  ph_a : Constant  Value=0
  ph_b : Constant  Value=-120
  ph_c : Constant  Value=120
  Out1 : Outport  VectorParamsAs1DForOutWhenUnconnected=off
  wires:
  Switch/1 -> Switch1/1
  Switch1/1 -> Out1/1
  Constant6/1 -> If/1
  If/1 -> If Action Subsystem/Action
  If/2 -> If Action Subsystem1/Action
  If/3 -> If Action Subsystem2/Action
  Demux/1 -> Switch/2
  Demux/2 -> Switch1/2
  If Action Subsystem2/1(Out1) -> Logical Operator/1
  Mux/1 -> [control]
  If Action Subsystem/1(Out1) -> Mux/1
  Logical Operator/1 -> Data Type Conversion/1
  [control] -> Demux/1
  Data Type Conversion/1 -> Mux/2
  Constant9/1 -> Product/1
  ph_a/1 -> Add/2
  Add/1 -> Rad->Deg.2/1
  Magnitude-Angle to Complex/1 -> Switch/1
  Add1/1 -> Rad->Deg.1/1
  ph_b/1 -> Add1/2
  Add2/1 -> Rad->Deg.3/1
  ph_c/1 -> Add2/2
  Constant7/1 -> Magnitude-Angle to Complex/1, Magnitude-Angle to Complex2/1, Magnitude-Angle to Complex1/1
  Product/1 -> Add2/1, Add1/1, Add/1
  Constant8/1 -> Product/2
  Magnitude-Angle to Complex1/1 -> Switch/3
  Magnitude-Angle to Complex2/1 -> Switch1/3
  Rad->Deg.2/1 -> Magnitude-Angle to Complex/2
  Rad->Deg.1/1 -> Magnitude-Angle to Complex1/2
  Rad->Deg.3/1 -> Magnitude-Angle to Complex2/2

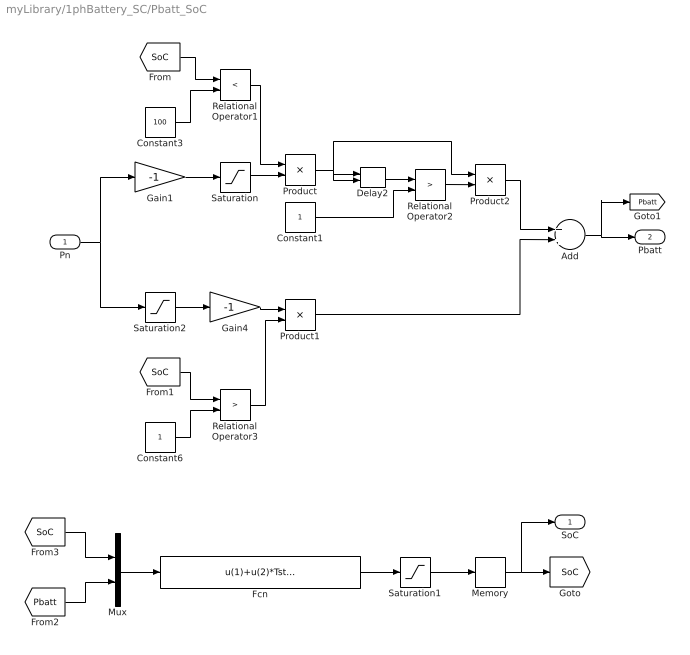
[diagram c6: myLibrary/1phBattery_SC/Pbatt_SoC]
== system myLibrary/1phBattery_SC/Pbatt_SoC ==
  Pn : Inport
  Add : Sum
  Constant1 : Constant
  Constant3 : Constant  Value=100
  Constant6 : Constant
  Delay2 : Delay  DelayLength=ch_delay  ExternalReset=Falling
  Fcn : Fcn  Expr=u(1)+u(2)*Tstep*100/(1e3*3600*Ecap)
  Gain1 : Gain  Gain=-1
  Gain4 : Gain  Gain=-1
  Memory : Memory  InitialCondition=SoC
  Mux : Mux  Inputs=2
  Product : Product
  Product1 : Product
  Product2 : Product
  Relational Operator1 : RelationalOperator  Operator=<  OutDataTypeStr=boolean  RndMeth=Simplest
  Relational Operator2 : RelationalOperator  Operator=>  OutDataTypeStr=boolean  RndMeth=Simplest
  Relational Operator3 : RelationalOperator  Operator=>  OutDataTypeStr=boolean  RndMeth=Simplest
  Saturation : Saturate  UpperLimit=Pch_max*1e3  LowerLimit=0
  Saturation1 : Saturate  UpperLimit=100  LowerLimit=0
  Saturation2 : Saturate  UpperLimit=Pdisc_max*1e3  LowerLimit=0
  SoC : Outport
  Pbatt : Outport  Port=2
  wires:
  Gain1/1 -> Saturation/1
  Pn/1 -> Gain1/1, Saturation2/1
  Saturation2/1 -> Gain4/1
  Memory/1 -> SoC/1, [SoC]
  [SoC] -> Relational Operator1/1
  Constant3/1 -> Relational Operator1/2
  [SoC] -> Relational Operator3/1
  Constant6/1 -> Relational Operator3/2
  Saturation/1 -> Product/2
  Relational Operator1/1 -> Product/1
  Gain4/1 -> Product1/1
  Relational Operator3/1 -> Product1/2
  Product1/1 -> Add/2
  Add/1 -> Pbatt/1, [Pbatt]
  [SoC] -> Mux/1
  [Pbatt] -> Mux/2
  Mux/1 -> Fcn/1
  Fcn/1 -> Saturation1/1
  Saturation1/1 -> Memory/1
  Constant1/1 -> Relational Operator2/2
  Delay2/1 -> Relational Operator2/1
  Product/1 -> Delay2/1, Product2/1, Delay2/2
  Product2/1 -> Add/1
  Relational Operator2/1 -> Product2/2

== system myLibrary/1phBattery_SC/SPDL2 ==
  P : Inport
  Q : Inport  Port=2
  Breaker : powerlib/Elements/Breaker  InitialState=1  SwitchingTimes=0  External=off  BreakerResistance=0.01  SnubberResistance=1e3  SnubberCapacitance=inf  Measurements=None  MoreParameters=on  NoBreakLoop=off
  Controlled Current Source : powerlib/Electrical Sources/Controlled Current Source  Initialize=on  Source_Type=AC  Amplitude=0  Phase=0  Frequency=50  Measurements=None
  Current Calculation : Subsystem
  Gain : Gain  Gain=sqrt(2)
  Initialization : Subsystem
  Snubber4 : powerlib/Elements/Series RLC Branch  LConnTagsString=__new0  RConnTagsString=__new0  BranchType=R  Resistance=1e6  Inductance=1e-3  SetiL0=off  InitialCurrent=0  Capacitance=1e-6  Setx0=off  InitialVoltage=0  Measurements=None
  Step : Step  Time=0.001  Before=-1  SampleTime=0
  Switch : Switch  Criteria=u2 > Threshold
  Voltage Measurement1 : powerlib/Measurements/Voltage Measurement  PhasorSimulation=off  OutputType=Complex  PSBequivalent=0
  Phase : PMIOPort  Side=Left
  Neutral : PMIOPort  Port=2  Side=Left
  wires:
  Switch/1 -> Current Calculation/1(Vp)
  Current Calculation/1(Isignal) -> [Icontrol]
  [Icontrol] -> Controlled Current Source/1
  Initialization/1(Out1) -> Gain/1
  Step/1 -> Switch/2
  Gain/1 -> Switch/3
  P/1 -> Current Calculation/2(P)
  Voltage Measurement1/1 -> [Vc]
  [Vc] -> Switch/1
  Q/1 -> Current Calculation/3(Q)
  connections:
  Neutral/RConn1 -- Snubber4/RConn1 -- Controlled Current Source/RConn1 -- Voltage Measurement1/LConn2
  Phase/RConn1 -- Breaker/RConn1 -- Controlled Current Source/LConn1 -- Voltage Measurement1/LConn1
  Snubber4/LConn1 -- Breaker/LConn1

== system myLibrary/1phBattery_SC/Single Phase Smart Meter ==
  Meas : Subsystem
  Phase-Ground Measurements : Subsystem
  Phase-Neutral Measurements : Subsystem
  Phase : PMIOPort  Side=Left
  Neutral : PMIOPort  Port=2  Side=Left
  p : PMIOPort  Port=3  Side=Right
  n : PMIOPort  Port=4  Side=Right
  Pout : Outport
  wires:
  Phase-Neutral Measurements/1(Vpn) -> Meas/1(Vpn)
  Phase-Ground Measurements/2(Ip_In) -> Meas/2(Ipn)
  Meas/1(P) -> Pout/1
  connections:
  Phase-Ground Measurements/LConn2 -- Phase-Neutral Measurements/LConn2 -- Neutral/RConn1
  Phase/RConn1 -- Phase-Neutral Measurements/LConn1 -- Phase-Ground Measurements/LConn1
  p/RConn1 -- Phase-Ground Measurements/RConn1
  n/RConn1 -- Phase-Ground Measurements/RConn2

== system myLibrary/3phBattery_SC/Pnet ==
  Mux2 : Mux  Inputs=3
  Three Phase Smart Meter : Subsystem
  Three-Phase V-I Measurement : powerlib/Measurements/Three-Phase V-I Measurement  VoltageMeasurement=no  SetLabelV=off  LabelV=Vabc  Vpu=off  VpuLL=off  CurrentMeasurement=yes  SetLabelI=off  LabelI=Iabc  Ipu=off  Pbase=100e6  Vbase=500e3  OutputType=Complex  PhasorSimulation=on  PSBequivalent=0
  Voltage Measurement1 : powerlib/Measurements/Voltage Measurement  PhasorSimulation=off  OutputType=Complex  PSBequivalent=0
  Voltage Measurement2 : powerlib/Measurements/Voltage Measurement  PhasorSimulation=off  OutputType=Complex  PSBequivalent=0
  Voltage Measurement4 : powerlib/Measurements/Voltage Measurement  PhasorSimulation=off  OutputType=Complex  PSBequivalent=0
  A : PMIOPort  Side=Left
  B : PMIOPort  Port=2  Side=Left
  C : PMIOPort  Port=3  Side=Left
  N : PMIOPort  Port=4  Side=Left
  a : PMIOPort  Port=5  Side=Right
  b : PMIOPort  Port=6  Side=Right
  c : PMIOPort  Port=7  Side=Right
  Pnet : Outport  VectorParamsAs1DForOutWhenUnconnected=off
  Qnet : Outport  Port=2  VectorParamsAs1DForOutWhenUnconnected=off
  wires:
  Three Phase Smart Meter/2(Qnet) -> Qnet/1
  Three-Phase V-I Measurement/1 -> Three Phase Smart Meter/2(Iabc)
  Three Phase Smart Meter/1(Pnet) -> Pnet/1
  Voltage Measurement2/1 -> Mux2/2
  Voltage Measurement1/1 -> Mux2/1
  Voltage Measurement4/1 -> Mux2/3
  Mux2/1 -> Three Phase Smart Meter/1(Vabc)
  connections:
  N/RConn1 -- Voltage Measurement4/LConn2 -- Voltage Measurement1/LConn2 -- Voltage Measurement2/LConn2
  C/RConn1 -- Voltage Measurement4/LConn1 -- Three-Phase V-I Measurement/LConn3
  A/RConn1 -- Voltage Measurement1/LConn1 -- Three-Phase V-I Measurement/LConn1
  B/RConn1 -- Voltage Measurement2/LConn1 -- Three-Phase V-I Measurement/LConn2
  c/RConn1 -- Three-Phase V-I Measurement/RConn3
  b/RConn1 -- Three-Phase V-I Measurement/RConn2
  a/RConn1 -- Three-Phase V-I Measurement/RConn1

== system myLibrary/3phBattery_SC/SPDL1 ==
  P : Inport
  Q : Inport  Port=2
  Breaker : powerlib/Elements/Breaker  InitialState=1  SwitchingTimes=0  External=off  BreakerResistance=0.01  SnubberResistance=1e3  SnubberCapacitance=inf  Measurements=None  MoreParameters=on  NoBreakLoop=off
  Controlled Current Source : powerlib/Electrical Sources/Controlled Current Source  Initialize=on  Source_Type=AC  Amplitude=0  Phase=0  Frequency=50  Measurements=None
  Current Calculation : Subsystem
  Gain : Gain  Gain=sqrt(2)
  Initialization : Subsystem
  Snubber4 : powerlib/Elements/Series RLC Branch  LConnTagsString=__new0  RConnTagsString=__new0  BranchType=R  Resistance=1e6  Inductance=1e-3  SetiL0=off  InitialCurrent=0  Capacitance=1e-6  Setx0=off  InitialVoltage=0  Measurements=None
  Step : Step  Time=0.001  Before=-1  SampleTime=0
  Switch : Switch  Criteria=u2 > Threshold
  Voltage Measurement1 : powerlib/Measurements/Voltage Measurement  PhasorSimulation=off  OutputType=Complex  PSBequivalent=0
  Phase : PMIOPort  Side=Left
  Neutral : PMIOPort  Port=2  Side=Left
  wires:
  Switch/1 -> Current Calculation/1(Vp)
  Current Calculation/1(Isignal) -> [Icontrol]
  [Icontrol] -> Controlled Current Source/1
  Initialization/1(Out1) -> Gain/1
  Step/1 -> Switch/2
  Gain/1 -> Switch/3
  P/1 -> Current Calculation/2(P)
  Voltage Measurement1/1 -> [Vc]
  [Vc] -> Switch/1
  Q/1 -> Current Calculation/3(Q)
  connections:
  Neutral/RConn1 -- Snubber4/RConn1 -- Controlled Current Source/RConn1 -- Voltage Measurement1/LConn2
  Phase/RConn1 -- Breaker/RConn1 -- Controlled Current Source/LConn1 -- Voltage Measurement1/LConn1
  Snubber4/LConn1 -- Breaker/LConn1

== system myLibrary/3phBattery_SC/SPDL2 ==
  P : Inport
  Q : Inport  Port=2
  Breaker : powerlib/Elements/Breaker  InitialState=1  SwitchingTimes=0  External=off  BreakerResistance=0.01  SnubberResistance=1e3  SnubberCapacitance=inf  Measurements=None  MoreParameters=on  NoBreakLoop=off
  Controlled Current Source : powerlib/Electrical Sources/Controlled Current Source  Initialize=on  Source_Type=AC  Amplitude=0  Phase=0  Frequency=50  Measurements=None
  Current Calculation : Subsystem
  Gain : Gain  Gain=sqrt(2)
  Initialization : Subsystem
  Snubber4 : powerlib/Elements/Series RLC Branch  LConnTagsString=__new0  RConnTagsString=__new0  BranchType=R  Resistance=1e6  Inductance=1e-3  SetiL0=off  InitialCurrent=0  Capacitance=1e-6  Setx0=off  InitialVoltage=0  Measurements=None
  Step : Step  Time=0.001  Before=-1  SampleTime=0
  Switch : Switch  Criteria=u2 > Threshold
  Voltage Measurement1 : powerlib/Measurements/Voltage Measurement  PhasorSimulation=off  OutputType=Complex  PSBequivalent=0
  Phase : PMIOPort  Side=Left
  Neutral : PMIOPort  Port=2  Side=Left
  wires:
  Switch/1 -> Current Calculation/1(Vp)
  Current Calculation/1(Isignal) -> [Icontrol]
  [Icontrol] -> Controlled Current Source/1
  Initialization/1(Out1) -> Gain/1
  Step/1 -> Switch/2
  Gain/1 -> Switch/3
  P/1 -> Current Calculation/2(P)
  Voltage Measurement1/1 -> [Vc]
  [Vc] -> Switch/1
  Q/1 -> Current Calculation/3(Q)
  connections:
  Neutral/RConn1 -- Snubber4/RConn1 -- Controlled Current Source/RConn1 -- Voltage Measurement1/LConn2
  Phase/RConn1 -- Breaker/RConn1 -- Controlled Current Source/LConn1 -- Voltage Measurement1/LConn1
  Snubber4/LConn1 -- Breaker/LConn1

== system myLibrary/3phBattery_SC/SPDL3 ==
  P : Inport
  Q : Inport  Port=2
  Breaker : powerlib/Elements/Breaker  InitialState=1  SwitchingTimes=0  External=off  BreakerResistance=0.01  SnubberResistance=1e3  SnubberCapacitance=inf  Measurements=None  MoreParameters=on  NoBreakLoop=off
  Controlled Current Source : powerlib/Electrical Sources/Controlled Current Source  Initialize=on  Source_Type=AC  Amplitude=0  Phase=0  Frequency=50  Measurements=None
  Current Calculation : Subsystem
  Gain : Gain  Gain=sqrt(2)
  Initialization : Subsystem
  Snubber4 : powerlib/Elements/Series RLC Branch  LConnTagsString=__new0  RConnTagsString=__new0  BranchType=R  Resistance=1e6  Inductance=1e-3  SetiL0=off  InitialCurrent=0  Capacitance=1e-6  Setx0=off  InitialVoltage=0  Measurements=None
  Step : Step  Time=0.001  Before=-1  SampleTime=0
  Switch : Switch  Criteria=u2 > Threshold
  Voltage Measurement1 : powerlib/Measurements/Voltage Measurement  PhasorSimulation=off  OutputType=Complex  PSBequivalent=0
  Phase : PMIOPort  Side=Left
  Neutral : PMIOPort  Port=2  Side=Left
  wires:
  Switch/1 -> Current Calculation/1(Vp)
  Current Calculation/1(Isignal) -> [Icontrol]
  [Icontrol] -> Controlled Current Source/1
  Initialization/1(Out1) -> Gain/1
  Step/1 -> Switch/2
  Gain/1 -> Switch/3
  P/1 -> Current Calculation/2(P)
  Voltage Measurement1/1 -> [Vc]
  [Vc] -> Switch/1
  Q/1 -> Current Calculation/3(Q)
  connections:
  Neutral/RConn1 -- Snubber4/RConn1 -- Controlled Current Source/RConn1 -- Voltage Measurement1/LConn2
  Phase/RConn1 -- Breaker/RConn1 -- Controlled Current Source/LConn1 -- Voltage Measurement1/LConn1
  Snubber4/LConn1 -- Breaker/LConn1

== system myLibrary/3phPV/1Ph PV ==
  Vp : Inport
  SPDL - Single Phase Dynamic Load (Phasor) : Subsystem  mask(Single-Phase Dynamic Load){Load_Profile=Load_Profile, Phase=Phase}
      mask prompts: Phase "Phase [A=1, B=2, C=3]"
      mask help: Single Phase Dynamic Load. The Load Profile is given by an external file.
  Phase : PMIOPort  Tag=PMCPort  Side=Left
  N : PMIOPort  Tag=PMCPort  Port=2  Side=Left
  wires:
  Vp/1 -> SPDL - Single Phase Dynamic Load (Phasor)/1(Vm_c)
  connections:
  N/RConn1 -- SPDL - Single Phase Dynamic Load (Phasor)/LConn2
  Phase/RConn1 -- SPDL - Single Phase Dynamic Load (Phasor)/LConn1

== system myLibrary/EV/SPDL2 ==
  P : Inport
  Q : Inport  Port=2
  Breaker : powerlib/Elements/Breaker  InitialState=1  SwitchingTimes=0  External=off  BreakerResistance=0.01  SnubberResistance=1e3  SnubberCapacitance=inf  Measurements=None  MoreParameters=on  NoBreakLoop=off
  Controlled Current Source : powerlib/Electrical Sources/Controlled Current Source  Initialize=on  Source_Type=AC  Amplitude=0  Phase=0  Frequency=50  Measurements=None
  Current Calculation : Subsystem
  Gain : Gain  Gain=sqrt(2)
  Snubber4 : powerlib/Elements/Series RLC Branch  LConnTagsString=__new0  RConnTagsString=__new0  BranchType=R  Resistance=1e6  Inductance=1e-3  SetiL0=off  InitialCurrent=0  Capacitance=1e-6  Setx0=off  InitialVoltage=0  Measurements=None
  Step : Step  Time=0.001  Before=-1  SampleTime=0
  Switch : Switch  Criteria=u2 > Threshold
  V Initialization : $bdroot/V Initialization  SystemSampleTime=-1  Latency=0  AutoFrameSizeCalculation=off
  Voltage Measurement1 : powerlib/Measurements/Voltage Measurement  PhasorSimulation=off  OutputType=Complex  PSBequivalent=0
  Phase : PMIOPort  Side=Left
  Neutral : PMIOPort  Port=2  Side=Left
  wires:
  Q/1 -> Current Calculation/3(Q)
  [Vc] -> Switch/1
  Voltage Measurement1/1 -> [Vc]
  P/1 -> Current Calculation/2(P)
  Gain/1 -> Switch/3
  Step/1 -> Switch/2
  V Initialization/1 -> Gain/1
  [Icontrol] -> Controlled Current Source/1
  Current Calculation/1(Isignal) -> [Icontrol]
  Switch/1 -> Current Calculation/1(Vp)
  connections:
  Snubber4/LConn1 -- Breaker/LConn1
  Voltage Measurement1/LConn1 -- Controlled Current Source/LConn1 -- Breaker/RConn1 -- Phase/RConn1
  Voltage Measurement1/LConn2 -- Controlled Current Source/RConn1 -- Snubber4/RConn1 -- Neutral/RConn1
